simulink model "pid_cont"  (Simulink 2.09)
settings: Solver=ode45  StartTime=0.0  StopTime=200.0  RelTol=1e-3  AbsTol=1e-6
undefined symbols (not defined in the file or in its folder): gamma, Kp, Td, Ti

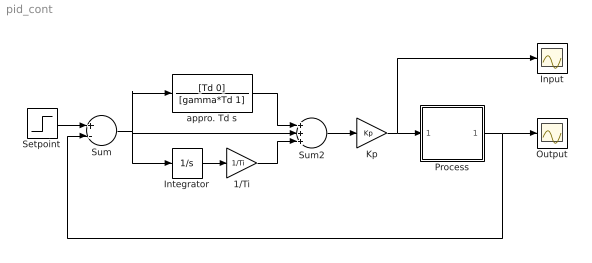
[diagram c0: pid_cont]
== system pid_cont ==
  1/Ti : Gain  Gain=1/Ti
  Input : Scope
  Integrator : Integrator  ExternalReset=none  InitialConditionSource=internal  InitialCondition=0  LimitOutput=off  UpperSaturationLimit=inf  LowerSaturationLimit=-inf  ShowSaturationPort=off  ShowStatePort=off  AbsoluteTolerance=auto
  Kp : Gain  Gain=Kp
  Output : Scope
  Process : Subsystem
  Setpoint : Step  Time=10  Before=0  After=10
  Sum : Sum  Inputs=+-
  Sum2 : Sum  Inputs=+++
  appro. Td s : TransferFcn  Numerator=[Td 0]  Denominator=[gamma*Td 1]
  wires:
  Kp/1 -> Input/1, Process/1(In1)
  Sum2/1 -> Kp/1
  Setpoint/1 -> Sum/1
  Process/1(Out1) -> Output/1, Sum/2
  1/Ti/1 -> Sum2/3
  Sum/1 -> Sum2/2, appro. Td s/1, Integrator/1
  appro. Td s/1 -> Sum2/1
  Integrator/1 -> 1/Ti/1

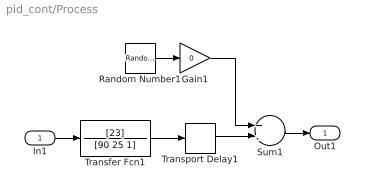
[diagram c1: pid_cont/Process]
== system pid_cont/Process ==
  In1 : Inport  Port=1  PortWidth=-1  SampleTime=-1
  Gain1 : Gain  Gain=0
  Random Number1 : RandomNumber  Mean=0  Variance=0.2  Seed=0  SampleTime=0
  Sum1 : Sum  Inputs=++
  Transfer Fcn1 : TransferFcn  Numerator=[23]  Denominator=[90 25 1]
  Transport Delay1 : TransportDelay  DelayTime=8  InitialInput=0  BufferSize=1024
  Out1 : Outport  Port=1  InitialOutput=0
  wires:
  Gain1/1 -> Sum1/1
  Random Number1/1 -> Gain1/1
  Transfer Fcn1/1 -> Transport Delay1/1
  Transport Delay1/1 -> Sum1/2
  Sum1/1 -> Out1/1
  In1/1 -> Transfer Fcn1/1
